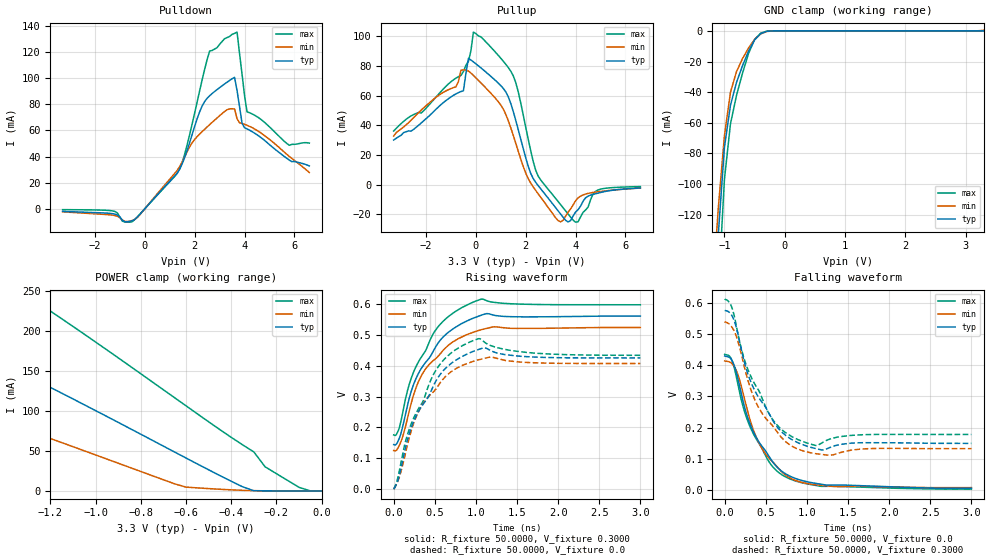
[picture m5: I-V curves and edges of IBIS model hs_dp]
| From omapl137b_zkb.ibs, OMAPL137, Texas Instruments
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|   Model hs_dp
[Model] hs_dp
Model_type   3-state
Polarity   Non-Inverting
Enable   Active-High
Vmeas =   0.2000V
C_comp   0.5000pF   0.4000pF   0.8000pF
[Temperature Range]   25.0000   0.1100k   -40.0000
[Voltage Range]   3.3000V   3.0000V   3.6000V
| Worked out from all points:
|   slope of the pulldown table from 0 to 0.495 V, typ, clamps not added: 46.8 ohm
|   slope of the pullup table from 0 to 0.495 V, typ, clamps not added: 71.7 ohm
|   GND clamp passes 1 mA (typ) near -0.35 V on its own axis
|   POWER clamp passes 1 mA (typ) near -0.31 V on its own axis
|   rising waveform, R_fixture 50.0000, V_fixture 0.3000: 20-80 % time 421ps typ, 438ps min, 385ps max; typ from 0.144 V to 0.561 V
|   rising waveform, R_fixture 50.0000, V_fixture 0.0: 20-80 % time 389ps typ, 404ps min, 352ps max; typ from 0 V to 0.425 V
|   falling waveform, R_fixture 50.0000, V_fixture 0.0: 20-80 % time 412ps typ, 386ps min, 389ps max; typ from 0.429 V to 0.007 V
|   falling waveform, R_fixture 50.0000, V_fixture 0.3000: 20-80 % time 390ps typ, 376ps min, 358ps max; typ from 0.575 V to 0.15 V
[Pulldown]
|Voltage   I(typ)   I(min)   I(max)
-3.3V     -2.051mA   -2.455mA   -732.7uA
-800mV    -10.03mA   -9.8mA     -10.22mA
-300mV    -6.393mA   -6.693mA   -6.262mA
1.4V      30.45mA    32.38mA    30.68mA
2.2V      74.38mA    57.27mA    90.59mA
2.6V      86.68mA    64.52mA    121mA
3.6V      100.8mA    76.52mA    134.5mA
3.7V      90.6mA     68.95mA    135.5mA
3.9V      65.59mA    65.37mA    103.2mA
4.1V      61.23mA    63.98mA    74.29mA
5.8V      37.26mA    40.06mA    48.64mA
6.6V      32.8mA     27.76mA    50.31mA
[Pullup]
|Voltage   I(typ)   I(min)   I(max)
-3.3V     29.98mA    32.67mA    36.06mA
-800mV    61.1mA     65.9mA     71.69mA
-600mV    62.66mA    77.07mA    73.54mA
-300mV    85.06mA    76.48mA    83mA
-100mV    82.68mA    73.55mA    102.8mA
1V        66.65mA    53.56mA    85.09mA
1.5V      49.2mA     33.12mA    73.24mA
2.4V      1.471mA    -3.982mA   9.583mA
3.2V      -15.62mA   -22.39mA   -9.409mA
3.9V      -21.25mA   -13.82mA   -23.98mA
4.9V      -5.814mA   -4.873mA   -3.67mA
6.6V      -2.327mA   -2.383mA   -1.391mA
[GND_clamp]
|Voltage   I(typ)   I(min)   I(max)
-3.3V     -2.102A    -1.576A    -3.228A
-1.2V     -207.9mA   -171.6mA   -289.7mA
-1.1V     -132.1mA   -115mA     -169.9mA
-1V       -76.03mA   -68.46mA   -96.96mA
-900mV    -48.63mA   -40.12mA   -60.78mA
-800mV    -33.68mA   -26.64mA   -42.17mA
-700mV    -22.71mA   -18.11mA   -27.61mA
-600mV    -13.24mA   -11.16mA   -14.78mA
-500mV    -5.931mA   -5.609mA   -5.62mA
-400mV    -1.814mA   -2.008mA   -1.538mA
-200mV    -13.57uA   -34.99uA   -6.398uA
3.3V      27.63uA    374.3uA    27.55uA
[POWER_clamp]
|Voltage   I(typ)   I(min)   I(max)
-3.3V     434.5mA    862.7mA    595.9mA
-2.35V    281.5mA    249.7mA    422.2mA
-2.2V     262.7mA    179.3mA    401.4mA
-2.1V     250.3mA    155mA      385.4mA
-2V       237.7mA    143.8mA    368.9mA
-1.3V     143.6mA    75.64mA    243.6mA
-600mV    41.12mA    4.791mA    106.3mA
-350mV    5.253mA    778.4uA    57.63mA
-300mV    274.5uA    374.3uA    48.71mA
-250mV    91.11uA    154.3uA    30.09mA
-100mV    28.77uA    28.48uA    4.516mA
0V        27.63uA    25.47uA    25.47uA
[Ramp]
| variable   typ   min   max
dV/dt_r   0.2551/0.3895n   0.2442/0.4044n   0.2602/0.3521n
dV/dt_f   17.9155m/0.4973n   34.0374m/0.4719n   8.2862m/28.1934p
R_load =   50.0000
[Rising Waveform]
R_fixture=   50.0000
V_fixture=   0.3000
V_fixture_min=  0.2700
V_fixture_max=  0.3600
|time   V(typ)   V(min)   V(max)
0s        144.4mV    125.2mV    175.8mV
51.05ps   154.4mV    132.5mV    186.6mV
96.1ps    187.8mV    159.1mV    229.2mV
201.2ps   305.8mV    265.9mV    349.6mV
273.3ps   359.4mV    329.6mV    397.9mV
351.4ps   397.4mV    374.6mV    433.8mV
546.5ps   475.7mV    432.2mV    528.1mV
849.8ps   539.7mV    496mV      591.3mV
1.132ns   568.7mV    521.3mV    610.5mV
3ns       560.9mV    523.8mV    597.4mV
[Rising Waveform]
R_fixture=   50.0000
V_fixture=   0.0
V_fixture_min=  0.0
V_fixture_max=  0.0
|time   V(typ)   V(min)   V(max)
0s        1.834uV    5.859uV    1.654uV
60.06ps   35.64mV    32.41mV    48.06mV
171.2ps   162.9mV    147.3mV    179.9mV
324.3ps   262mV      262.2mV    270.3mV
540.5ps   362.2mV    334.7mV    396.3mV
831.8ps   429.9mV    400.6mV    464.5mV
1.033ns   452.8mV    419.3mV    487.6mV
1.105ns   457.8mV    424.2mV    476.2mV
1.655ns   428.7mV    410.2mV    442.1mV
3ns       425.2mV    407mV      433.7mV
[Falling Waveform]
R_fixture=   50.0000
V_fixture=   0.0
V_fixture_min=  0.0
V_fixture_max=  0.0
|time   V(typ)   V(min)   V(max)
0s        429.2mV    413.4mV    434.5mV
81.08ps   418mV      406.6mV    419.5mV
144.1ps   374.1mV    380.9mV    359.3mV
231.2ps   275.6mV    302.1mV    260.1mV
336.3ps   193.8mV    201.8mV    187mV
489.5ps   128.6mV    118.9mV    113.8mV
732.7ps   53.84mV    50.28mV    43.72mV
939.9ps   31.23mV    25.17mV    23.87mV
1.315ns   17.04mV    12.43mV    12.76mV
3ns       6.544mV    8.556mV    3.719mV
[Falling Waveform]
R_fixture=   50.0000
V_fixture=   0.3000
V_fixture_min=  0.2700
V_fixture_max=  0.3600
|time   V(typ)   V(min)   V(max)
0s        575mV      539.2mV    611.2mV
69.07ps   565.5mV    528mV      595.5mV
123.1ps   536.5mV    504.4mV    549.4mV
207.2ps   443.9mV    429.4mV    447mV
297.3ps   360.2mV    338.6mV    376.2mV
510.5ps   259.7mV    226.4mV    259.2mV
822.8ps   161mV      140.2mV    170.6mV
1.186ns   128.8mV    114.1mV    152.3mV
1.619ns   151.7mV    130.8mV    176.8mV
3ns       149.9mV    133mV      178.4mV
